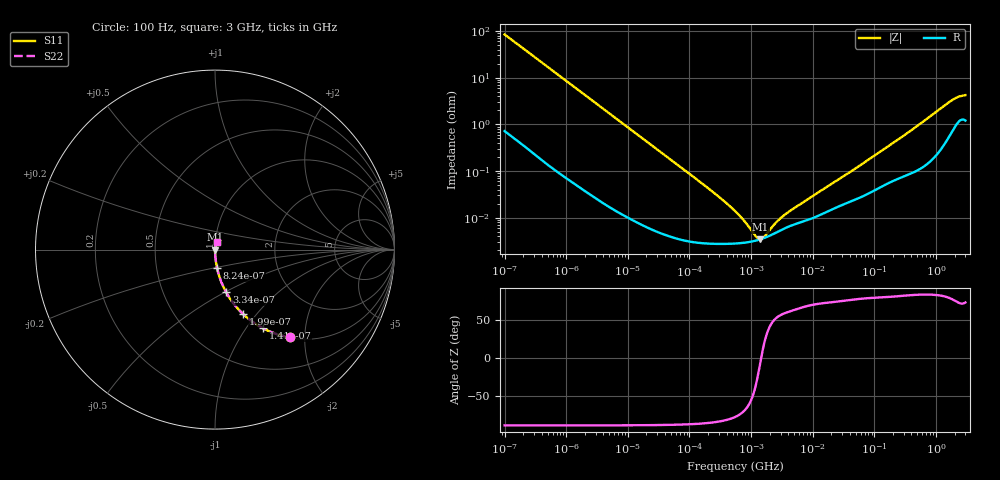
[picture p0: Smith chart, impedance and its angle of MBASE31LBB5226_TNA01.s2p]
! MBASE31LBB5226_TNA01  S-PARAMETER MODEL  ( Standard Model )
! Model Generated by TAIYO YUDEN Corporation (http://www.ty-top.com)
! Version 1.0
! TAIYO YUDEN Control No. 220601
! Copyright(c) 2012 TAIYO YUDEN CO.,LTD. All Rights Reserved.
! Product Description (link to TY-COMPAS)
! https://ds.yuden.co.jp/TYCOMPAS/or/detail?pn=MBASE31LBB5226MTNA01&u=M
! Products Name : Multilayer Ceramic Capacitors
! Characteristics :
!  Capacitance : 22 [uF] , Rated Voltage : 16 [V] , TCC : X5R
!  Case Size : 3.2 x 1.6 / 0.126 x 0.063 [mm/inch] , Thickness : 1.6 / 0.063 [mm/inch]
!  (Conditions: Temperature = 25 [degC] , DC Bias Voltage = 0 [V])
! External Node Assignments :
!  1  o---| |---o  2
! GND o---------o GND
! Frequency Range : 100Hz  -  3GHz  [ 401 STEP ]
# MHZ S RI R 50
! Freq[MHz].  S11 Real  S11 Imag  S21 Real  S21 Imag  S12 Real  S12 Imag  S22 Real  S22 Imag
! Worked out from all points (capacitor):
!   401 points, 100 Hz to 3 GHz, reference 50 ohm
!   read as one part in series: C = 18.8 uF near 109 Hz
!   lowest |Z| = 3.46 mohm at 1.412 MHz (marker M1)
!   series resonance near 1.458 MHz, so ESL is about 630 pH
!   S11 on the Smith chart (normalised r, x): 100 Hz: 1.01, -1.69; 141 Hz: 1.01, -1.20; 199 Hz: 1.01, -0.85; 334 Hz: 1.00, -0.51; 824 Hz: 1.00, -0.21; 3 GHz: 1.02, +0.08
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0.0001  0.4169 -0.4888  0.5831 0.4888  0.5831 0.4888  0.4169 -0.4888
0.000141  0.2661 -0.4377  0.7339 0.4377  0.7339 0.4377  0.2661 -0.4377
0.000199  0.1555 -0.3582  0.8445 0.3582  0.8445 0.3582  0.1555 -0.3582
0.000334  0.0626 -0.2382  0.9374 0.2382  0.9374 0.2382  0.0626 -0.2382
0.000513  0.028 -0.1611  0.972 0.1611  0.972 0.1611  0.028 -0.1611
0.000824  0.0114 -0.1023  0.9886 0.1023  0.9886 0.1023  0.0114 -0.1023
0.001788  0.0027 -0.0478  0.9973 0.0478  0.9973 0.0478  0.0027 -0.0478
0.005476  0.000405 -0.0157  0.9996 0.0157  0.9996 0.0157  0.000405 -0.0157
0.031977  5.54e-05 -0.00272  0.9999 0.00272  0.9999 0.00272  5.54e-05 -0.00272
0.231582  2.78e-05 -0.000369  1 0.000369  1 0.000369  2.78e-05 -0.000369
0.547723  2.8e-05 -0.000137  1 0.000137  1 0.000137  2.8e-05 -0.000137
0.650627  2.84e-05 -0.000107  1 0.000107  1 0.000107  2.84e-05 -0.000107
0.740304  2.89e-05 -8.69e-05  1 8.69e-05  1 8.69e-05  2.89e-05 -8.69e-05
1.411895  3.44e-05 -3.66e-06  1 3.66e-06  1 3.66e-06  3.44e-05 -3.66e-06
3.063887  5.43e-05 8.39e-05  0.9999 -8.39e-05  0.9999 -8.39e-05  5.43e-05 8.39e-05
9.794414  9.71e-05 0.000269  0.9999 -0.000269  0.9999 -0.000269  9.71e-05 0.000269
44.18008  0.000231 0.00101  0.9998 -0.00101  0.9998 -0.00101  0.000231 0.00101
175.1444  0.000574 0.00348  0.9994 -0.00348  0.9994 -0.00348  0.000574 0.00348
414.2403  0.000972 0.00771  0.999 -0.00771  0.999 -0.00771  0.000972 0.00771
1789.813  0.00765 0.0314  0.9923 -0.0314  0.9923 -0.0314  0.00765 0.0314
2317.205  0.0125 0.0365  0.9875 -0.0365  0.9875 -0.0365  0.0125 0.0365
3000  0.0135 0.0396  0.9865 -0.0396  0.9865 -0.0396  0.0135 0.0396
